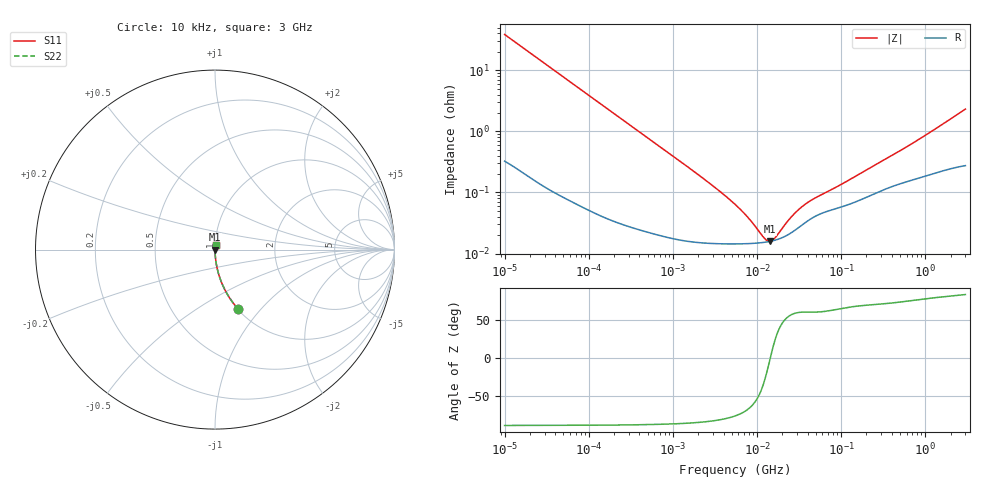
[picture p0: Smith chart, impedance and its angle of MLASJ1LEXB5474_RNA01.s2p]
! MLASJ1LEXB5474_RNA01  S-PARAMETER MODEL  ( Standard Model )
! Model Generated by TAIYO YUDEN Corporation (http://www.ty-top.com)
! Version 1.0
! TAIYO YUDEN Control No. 220601
! Copyright(c) 2015 TAIYO YUDEN CO.,LTD. All Rights Reserved.
! Product Description (link to TY-COMPAS)
! https://ds.yuden.co.jp/TYCOMPAS/or/detail?pn=MLASJ1LEXB5474KRNA01&u=M
! Products Name : Multilayer Ceramic Capacitors
! Characteristics :
!  Capacitance : 0.47 [uF] , Rated Voltage : 6.3 [V] , TCC : X5R
!  Case Size : 1.0 x 0.5 / 0.039 x 0.02 [mm/inch] , Thickness : 0.18 / 0.007 [mm/inch]
!  (Conditions: Temperature = 25 [degC] , DC Bias Voltage = 0 [V])
! External Node Assignments :
!  1  o---| |---o  2
! GND o---------o GND
! Frequency Range : 10kHz  -  3GHz  [ 401 STEP ]
# MHZ S RI R 50
! Freq[MHz].  S11 Real  S11 Imag  S21 Real  S21 Imag  S12 Real  S12 Imag  S22 Real  S22 Imag
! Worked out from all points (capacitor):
!   401 points, 10 kHz to 3 GHz, reference 50 ohm
!   read as one part in series: C = 413 nF near 10.65 kHz
!   lowest |Z| = 15.8 mohm at 14.1 MHz (marker M1)
!   series resonance near 14.42 MHz, so ESL is about 290 pH
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0.01  0.1309 -0.3331  0.8691 0.3331  0.8691 0.3331  0.1309 -0.3331
0.016047  0.0564 -0.2263  0.9436 0.2263  0.9436 0.2263  0.0564 -0.2263
0.027426  0.0207 -0.1379  0.9793 0.1379  0.9793 0.1379  0.0207 -0.1379
0.045421  0.0081 -0.0846  0.9919 0.0846  0.9919 0.0846  0.0081 -0.0846
0.082683  0.00279 -0.0469  0.9972 0.0469  0.9972 0.0469  0.00279 -0.0469
0.683653  0.000232 -0.00576  0.9998 0.00576  0.9998 0.00576  0.000232 -0.00576
2.652321  0.000149 -0.00145  0.9999 0.00145  0.9999 0.00145  0.000149 -0.00145
5.477226  0.000144 -0.000623  0.9999 0.000623  0.9999 0.000623  0.000144 -0.000623
7.996027  0.000146 -0.000346  0.9999 0.000346  0.9999 0.000346  0.000146 -0.000346
12.04705  0.000152 -0.000101  0.9998 0.000101  0.9998 0.000101  0.000152 -0.000101
13.24217  0.000155 -4.76e-05  0.9998 4.76e-05  0.9998 4.76e-05  0.000155 -4.76e-05
14.10408  0.000158 -1.23e-05  0.9998 1.23e-05  0.9998 1.23e-05  0.000158 -1.23e-05
15.02209  0.000161 2.29e-05  0.9998 -2.29e-05  0.9998 -2.29e-05  0.000161 2.29e-05
16.51234  0.000166 7.59e-05  0.9998 -7.59e-05  0.9998 -7.59e-05  0.000166 7.59e-05
23.35767  0.000203 0.000277  0.9998 -0.000277  0.9998 -0.000277  0.000203 0.000277
29.12589  0.000248 0.00041  0.9998 -0.00041  0.9998 -0.00041  0.000248 0.00041
36.31858  0.000311 0.000539  0.9997 -0.000539  0.9997 -0.000539  0.000311 0.000539
45.28751  0.000382 0.000659  0.9996 -0.000659  0.9996 -0.000659  0.000382 0.000659
102.7996  0.000585 0.00125  0.9994 -0.00125  0.9994 -0.00125  0.000585 0.00125
374.4521  0.00121 0.00362  0.9988 -0.00362  0.9988 -0.00362  0.00121 0.00362
823.6  0.00175 0.00703  0.9982 -0.00703  0.9982 -0.00703  0.00175 0.00703
3000  0.00326 0.0228  0.9967 -0.0228  0.9967 -0.0228  0.00326 0.0228
